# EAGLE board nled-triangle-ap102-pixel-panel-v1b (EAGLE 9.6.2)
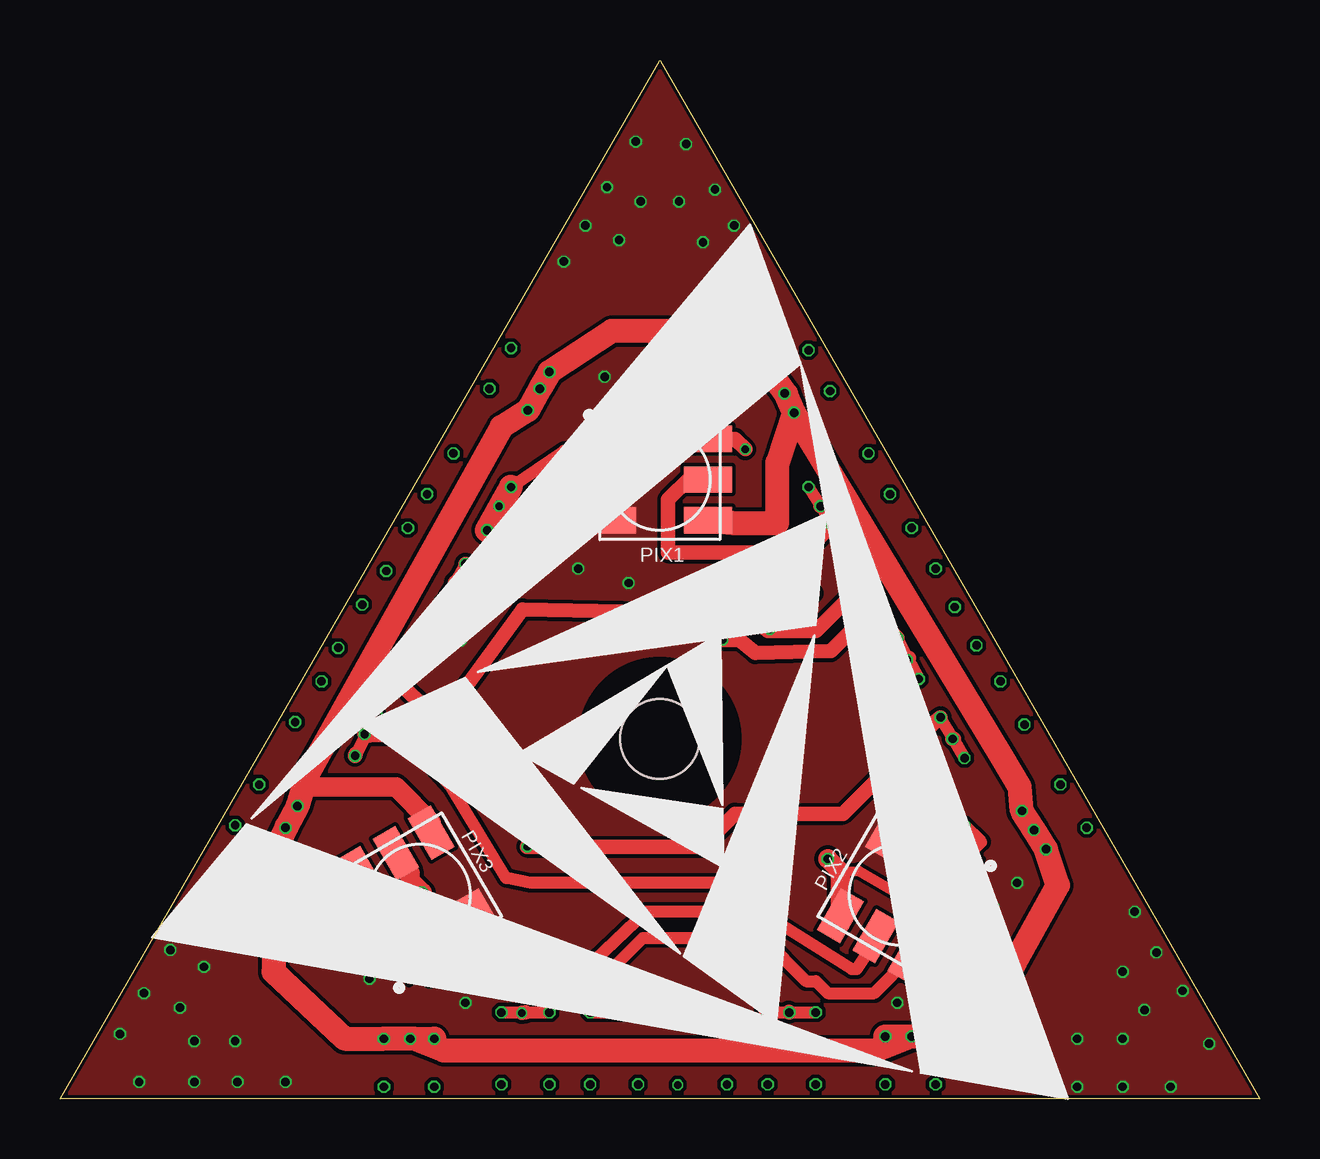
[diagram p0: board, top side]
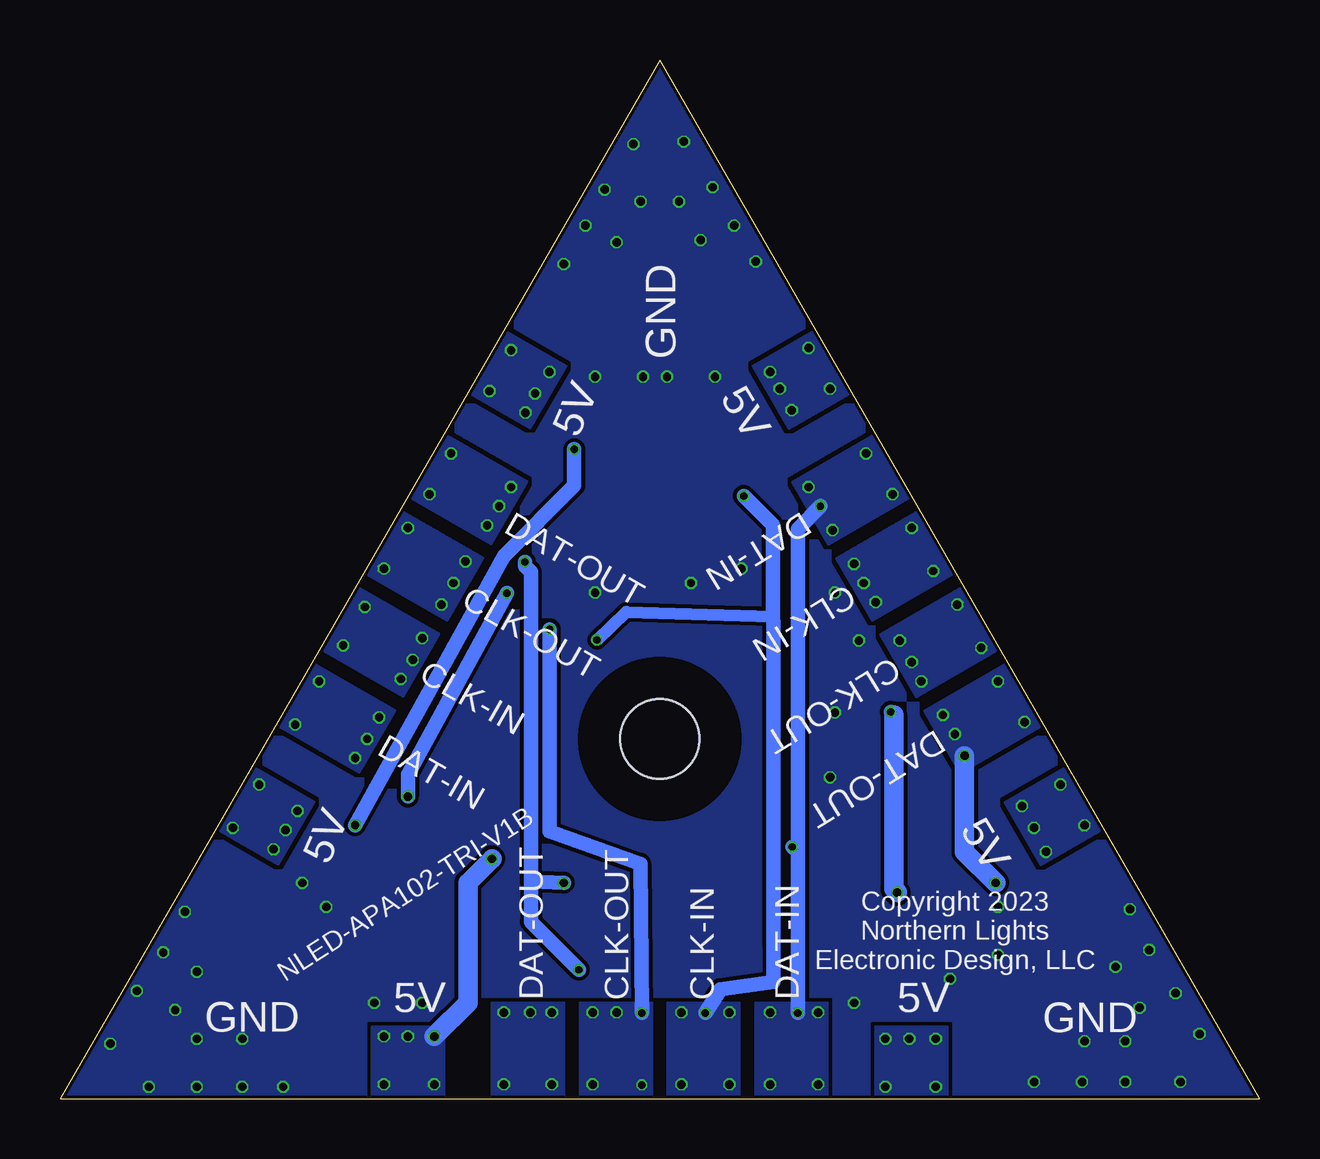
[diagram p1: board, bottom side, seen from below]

Size 50 x 43.3 mm. Coordinates in mm from the lower left corner, seen from the top.
Outline: 25,43.3 50,0 0,0 25,43.3
Copper layers (1*16): Top 0.035mm / dielectric 1.6mm / Bottom 0.035mm
Design rules "nled-2layer *": minimum track width 6mil, minimum drill 0.3mm, track to track 6mil, track to pad 6mil, pad to pad 6mil, via to via 6mil, smd to smd 6mil, copper to edge 0.15mm, drill to drill 6mil, minimum pad ring 10mil, minimum via ring 3mil, stop-mask expansion 4mil, vias tented up to drill 100mil, thermal gap 10mil
Net classes: 0 default: width 0.61 mm
Holes 3.3 mm at 25,15
tRestrict: area 21.8,11.8 to 28.2,18.2
bRestrict: area 21.8,11.8 to 28.2,18.2

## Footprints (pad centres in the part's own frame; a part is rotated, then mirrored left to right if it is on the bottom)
APA102_5050 = smd 2 x 1.1: 1 -2,1.7; 2 -2,0; 3 -2,-1.7; 4 2,-1.7; 5 2,0; 6 2,1.7

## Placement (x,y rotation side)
PIX1  APA102-V2  [APA102_5050]  25,25.81 0 top
PIX2  APA102-V2  [APA102_5050]  35,8.51 240 top
PIX3  APA102-V2  [APA102_5050]  15,8.51 120 top

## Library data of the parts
PIX1-PIX3 = NLED-optoelectric

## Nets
CLK-IN: PIX1.2
CLK-OUT: PIX3.5
DAT-IN: PIX1.1
DAT-OUT: PIX3.6
GND: PIX1.3 PIX2.3 PIX3.3
N$1: PIX1.6 PIX2.1
N$2: PIX1.5 PIX2.2
N$6: PIX2.6 PIX3.1
N$7: PIX2.5 PIX3.2
VCC: PIX1.4 PIX2.4 PIX3.4

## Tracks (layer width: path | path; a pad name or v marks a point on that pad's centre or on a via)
CLK-IN  (via drill 0.3, 0.35)
  Top 0.508: v16,20.7 16.46,21.52 v16.9,22.3 | v22.1,3.6 23.1,3.6 | 23.12,3.6 v24.1,3.6 | v35.8,17.5 35.34,18.36 v34.9,19.2
  Top 0.61: v35.3,18.3 35.38,18.38 35.34,18.36 | v16.5,21.5 16.46,21.52 | PIX1.2 23,25.88 22.25,25.88 v21.5,25.12 21.38,24.88 18.75,22.25 17.12,22.25 v16.9,22.3 | v34.9,19.2 34.37,19.73 33.2,19.73 32.13,18.66 28.99,18.58 28.32,19.12 v27.62,19.12
  Bottom 0.508: v27.62,19.12 26.4,20.3 20.29,20.1
  Bottom 0.61: v23.1,3.58 22.48,4.56 20.26,4.87 20.27,6.41 20.27,19.81 20.29,20.1 20.29,23.91 v21.5,25.12
  other vias: 22.1,0.6 24.1,0.6 38.2,18.9 37.3,20.5 14.5,23.8 13.6,22
  pour Bottom: 24.67,0 21.67,0 21.67,4 24.67,4
  pour Bottom: 37.67,21.37 39.17,18.77 35.7,16.77 34.2,19.37
  pour Bottom: 12.68,21.93 14.18,24.53 17.64,22.53 16.14,19.93
CLK-OUT  (via drill 0.3, 0.35)
  Top 0.508: v14.1,17.4 14.54,18.23 v15,19.1 | 25.8,3.6 v26.8,3.6 26.88,3.6 v27.8,3.6 | v33.1,22.4 v33.6,21.5 v33.61,21.49 v34.1,20.6
  Top 0.61: v26.8,3.6 26.88,3.62 26.88,3.6 | v33.61,21.49 33.62,21.5 v33.6,21.5 33.38,21.38 31.5,19.5 29.59,19.5 | v14.5,18.2 14.5,18.25 14.54,18.23 | v14.1,17.4 v15.38,16.12 16.32,16.35 19.27,20.4 28.7,20.2 29.5,19.5 29.59,19.5 | v29.59,19.57 29.59,19.5
  Top 0.813: PIX3.5 14,10 14.6,9.4 14.6,9.1 v15.1,8.6
  Bottom 0.61: v15.38,16.12 15.25,16 | v25.75,3.58 25.8,9.79 29.59,11.15 v29.59,19.57
  Bottom 0.813: 15.25,16 15.25,8.75 v15.1,8.6
  other vias: 25.75,0.57 27.8,0.6 36.5,22.1 35.5,23.8 12.6,20.6 11.6,18.8
  pour Bottom: 28.33,0 25.33,0 25.33,4 28.33,4
  pour Bottom: 35.83,24.55 37.33,21.95 33.87,19.95 32.37,22.54
  pour Bottom: 10.84,18.75 12.34,21.35 15.81,19.35 14.31,16.75
DAT-IN  (via drill 0.3, 0.35)
  Top 0.508: v18.8,25.5 21,27 PIX1.1 | v18.4,3.6 19.4,3.6 v20.4,3.6 | v37.7,14.2 37.23,14.99 v36.7,15.9
  Top 0.61: v37.2,15 37.25,15 37.23,14.99 | v19.25,3.58 19.4,3.6 | v19.48,10.5 26.75,10.5 28.12,11.88 32.62,11.88 36.5,15.75 v36.7,15.9
  Top 1: v17.8,23.7 v18.8,25.5
  Bottom 0.61: 19.25,10.43 19.25,23.75 v18.3,24.7 | 19.25,10.43 v19.25,3.58 | v19.48,10.5 19.41,10.43 19.25,10.43
  other vias: 18.4,0.6 20.4,0.6 40.2,15.6 39.2,17.4 16.4,26.9 15.3,25.2
  pour Bottom: 21,0 18,0 18,4 21,4
  pour Bottom: 39.5,18.19 41,15.6 37.54,13.6 36.04,16.19
  pour Bottom: 14.51,25.1 16.01,27.7 19.47,25.7 17.97,23.1
DAT-OUT  (via drill 0.3, 0.35)
  Top 0.508: 12.79,15.23 v12.3,14.3 | 12.79,15.23 v13.2,16 | v29.5,3.6 30.38,3.6 v30.4,3.6 v31.5,3.6 | v31.2,25.5 31.69,24.71 v31.7,24.7 v32.2,23.9 | v29,9 19.6,9 18.6,9.2 16.3,13 14.4,15.1 12.92,15.1 12.79,15.23
  Top 0.61: v12.7,15.2 12.75,15.25 12.79,15.23 | v31.7,24.7 31.75,24.75 31.69,24.71 | v30.4,3.6 30.38,3.62 30.38,3.6 | v29.5,3.6 29.38,3.75 29.36,4.56 29.36,4.57 v28.38,5.38 | v30.62,22.38 32,23.75 v32.2,23.9 | 12.32,14.38 v12.3,14.3
  Top 0.813: PIX3.6 11.39,9.39 v11,9
  Bottom 0.61: v30.62,22.38 30.62,22.2 30.38,21.95 30.38,9.06 | 30.38,9.06 30.38,7.38 v28.38,5.38 | v29,9 30.38,9.06
  Bottom 0.813: v12.3,14.3 12.3,10.3 v11,9
  other vias: 29.5,0.6 31.5,0.6 34.6,25.2 33.7,26.9 9.8,15.7 10.9,17.4
  pour Bottom: 32,0 29,0 29,4 32,4
  pour Bottom: 34,27.72 35.5,25.12 32.04,23.12 30.54,25.72
  pour Bottom: 9.01,15.58 10.51,18.18 13.97,16.18 12.47,13.58
GND  (via drill 0.35)
  other vias: 6,5.5 5,3.8 5.6,2.4 7.3,2.4 45.2,3.7 44.3,5.3 44.3,2.5 42.4,2.5 25.8,37.4 26.8,35.7 24.2,37.4 23.3,35.8 10.9,8 10.9,6 12.9,5 38.9,8 39.9,9 22.7,30.1 24.7,30.1 25.7,30.1 27.7,30.1 17.7,16.1 17.9,13.4 27.7,21.1 34.9,4 40.7,0.5 44.3,0.5 42.4,0.5 46.3,0.5 46.8,4.5 45.7,6.1 44.8,7.8 47.9,2.3 21,34.9 21.9,36.4 22.8,38 27.3,37.9 28.1,36.4 29,34.8 26.1,39.8 24,39.9 5.4,7.9 9.4,0.7 7.4,0.7 5.6,0.7 3.5,4.4 4.6,6.2 2.5,2.7 3.3,0.7 17.7,21.1 16.7,19.1 21.6,22.1 23.7,21.5 16.9,4 36.9,4
  pour Bottom (no thermals): 5.2,3 7.6,7.16 5,8.66 1.73,3 0,0 3.46,0 10,0 10,3
  pour Bottom: 44.8,3 42.4,7.16 45,8.66 48.27,3 50,0 46.54,0 40,0 40,3
  pour Bottom: 25,37.3 27.4,33.14 30,34.64 26.73,40.3 25,43.3 23.27,40.3 20,34.64 22.6,33.14
  pour Bottom (rank 2, no thermals): 0,0 51,0 25,43
  pour Top (rank 2, no thermals): 0,0 51,0 25,43
N$1  (via drill 0.3, 0.35)
  Top 0.508: PIX2.1 37.47,9.77 38.4,10.7 v37.7,11.4
  Top 0.61: v28.57,27.07 28.14,27.5 PIX1.6
  Bottom 0.61: v28.57,27.07 28.57,25.56 31.5,22.62 v37.7,11.4
N$2  (via drill 0.3, 0.35)
  Top 0.508: PIX2.2 36,10.7 36.5,11.2 36.5,12.3 35.6,12.4 v35.5,12.6
  Top 0.61: v31.37,21.07 30.71,21.07 29,22.78 25.34,22.78 25.34,24.97 26.25,25.88 27,25.88 PIX1.5
  Bottom 0.61: v35.5,12.6 35.5,13.52 v31.37,21.07
N$6
  Top 0.508: PIX3.1 14.53,5.87 15.4,5 22.6,5 24.3,6.7 29.3,6.7 31.1,4.9 31.5,4.9 32,4.4 33.94,4.4 PIX2.6
N$7
  Top 0.508: PIX3.2 16,6.7 16.9,5.8 22.3,5.8 24.4,7.8 29.2,7.8 33,5.4 33.2,5.4 34,6.6 PIX2.5
VCC  (via drill 0.35)
  Top 0.406: 32.53,9.47 33.3,9.5 39.83,5.71
  Top 0.61: v9.4,11.3 9.38,11.38 9.45,11.34 | v20,29.6 20,29.62 20.02,29.62 | v40.6,11.2 40.62,11.25 40.59,11.22 | v30.2,29.4 30.25,29.38 30.26,29.38
  Top 0.813: PIX3.4 15.47,11.53 14,13 10.25,13 10.1,12.85 | PIX2.4 32.53,9.47 v32,10
  Top 1: 14.74,2.5 v15.6,2.5 | 14.74,2.5 v14.6,2.5 v13.5,2.5 11.87,2.5 8.9,5.3 v8.9,10.3 9.45,11.34 9.45,11.35 v9.9,12.2 10.1,12.85 10.3,13.5 18.4,28 v19.5,28.7 20.02,29.62 v20.4,30.3 23,32 28,32 v29.6,30.3 30.26,29.38 v30.6,28.6 | v34.4,2.6 v35.5,2.6 | v35.5,2.6 v36.5,2.6 38.1,2.6 39.83,5.71 41.6,8.9 v41.1,10.4 v40.6,11.2 40.59,11.22 v40.1,12 40,13 39.27,14.23 v30.6,28.6 | v30.6,28.6 29.9,26.5 29.9,24 28,24 PIX1.4 | v35.5,2.6 34,2 16,2 14.74,2.5
  Bottom 0.813: v34.4,2.6 33,4 33,9 v32,10
  other vias: 13.5,0.5 15.6,0.5 34.4,0.6 36.5,0.6 42.8,11.3 41.7,13.1 32.1,29.5 31.2,31.2 18.8,31.3 17.9,29.6 8.3,13.1 7.3,11.4
  pour Bottom: 6.51,11.25 8.01,13.85 10.61,12.35 9.11,9.75
  pour Bottom: 37,0 34,0 34,3 37,3
  pour Bottom: 16,0 13,0 13,3 16,3
  pour Bottom: 42,13.86 43.5,11.27 40.9,9.77 39.4,12.36
  pour Bottom: 31.5,32.05 33,29.45 30.4,27.95 28.9,30.55
  pour Bottom: 17.01,29.43 18.51,32.03 21.11,30.53 19.61,27.93

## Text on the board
bNames: GND | 5V | 5V | DAT-OUT / CLK-OUT / CLK-IN / DAT-IN | DAT-OUT / CLK-OUT / CLK-IN / DAT-IN | 5V | 5V | NLED-APA102-TRI-V1B | Copyright 2023 / Northern Lights / Electronic Design, LLC | 5V | DAT-OUT / CLK-OUT / CLK-IN / DAT-IN | 5V | GND | GND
